TYPE STR_AO :
STRUCT
MFC1_Flow_Setpoint	,
MFC1_Rate_Setpoint	,
LID_Temp_SV	,	//E02
Chamber_Temp1_SV	,//E06
Chamber_Temp2_SV	,//E07
Chamber_Temp3_SV	,//E08
AV102_Temp_SV	,//E14
AV101_Temp_SV	,//E15
AV104_Temp_SV	,//E16
AV105_Temp_SV	,
Exhaust1_3_Temp_SV	,//E14
Exhaust4_7_Temp_SV	,//E15
VG101_Pipe_Temp_SV	,//E16
Gate_Valve_Temp_SV	,//E18
APC_Temp_SV	,//E01
Stage_Temp1_SV	,
Stage_Temp2_SV	,
Stage_Temp3_SV	,
Stage_Temp4_SV	:REAL;

APC:VAT_OUT;

TMP:TMP_OUT;
END_STRUCT
END_TYPE
